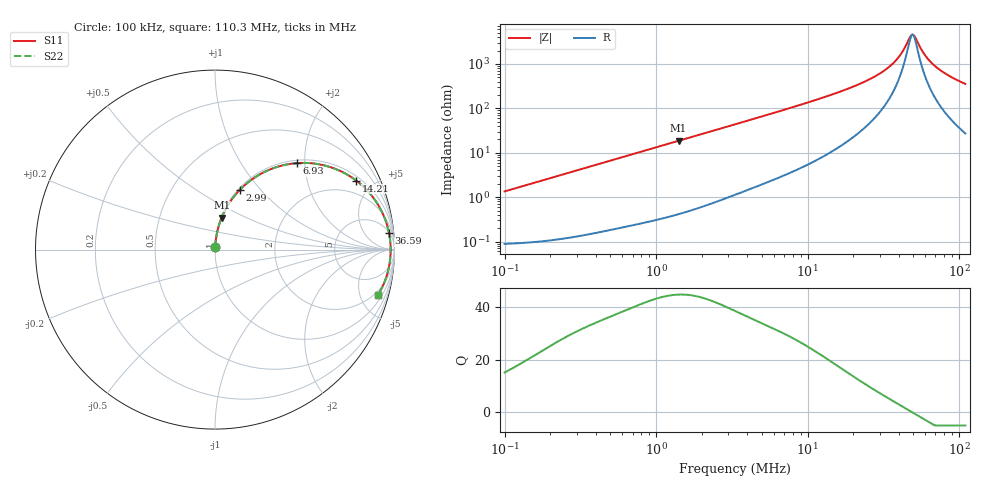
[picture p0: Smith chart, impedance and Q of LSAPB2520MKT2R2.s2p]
! LSAPB2520MKT2R2  S-PARAMETER MODEL  ( General Type )
! Model Generated by TAIYO YUDEN Corporation (http://www.ty-top.com)
! Version 2.0
! TAIYO YUDEN Control No. 20210629
! Copyright(c) 2015 TAIYO YUDEN CO.,LTD. All Rights Reserved.
! Product Description (link to TY-COMPAS)
! https://ds.yuden.co.jp/TYCOMPAS/or/detail?pn=LSAPB2520MKT2R2M&u=M
! Products Name : Inductors
! Characteristics :
!  Inductance : 2.2 uH , SRF(min) : -Hz , DC Resistance(max) : 0.09 Ohm
!  Rated Current : Saturation :2800 mA , Temp Rise : 2200 mA (40 degC)
!  Case Size : 2.5 x 2.0 / 0.098 x 0.079 [mm/inch] , Thickness : 1.2 / 0.047 [mm/inch]
!  (Conditions: Temperature = 25 degC , DC Bias Current/Voltage = 0A / 0V)
! External Node Assignments :
!  1  o---GGG---o  2
! GND o---------o GND
! Frequency Range : 0.1MHz  -  110.285862MHz  [ 402 STEP ]
# MHz S RI R 50
! Freq[MHz].  S11 Real  S11 Imag  S21 Real  S21 Imag  S12 Real  S12 Imag  S22 Real  S22 Imag
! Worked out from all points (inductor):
!   401 points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, 100 kHz to 110.3 MHz, reference 50 ohm
!   read as one part in series: L = 2.14 uH near 103.6 kHz
!   highest Q = 44.9 at 1.408 MHz (marker M1), where L = 2.1 uH
!   self-resonance near 49.28 MHz
!   S11 on the Smith chart (normalised r, x): 100 kHz: 1.00, +0.03; 2.99 MHz: 1.02, +0.79; 6.93 MHz: 1.06, +1.83; 14.21 MHz: 1.20, +3.98; 36.59 MHz: 6, +20; 110.3 MHz: 1.54, -7.08
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0.1  0.00107 0.0134  0.9989 -0.0134  0.9989 -0.0134  0.00107 0.0134
0.323312  0.00322 0.0431  0.9968 -0.0431  0.9968 -0.0431  0.00322 0.0431
1.045308  0.0217 0.1347  0.9783 -0.1347  0.9783 -0.1347  0.0217 0.1347
1.407833  0.037 0.178  0.963 -0.178  0.963 -0.178  0.037 0.178
2.989662  0.1397 0.3344  0.8603 -0.3344  0.8603 -0.3344  0.1397 0.3344
3.320932  0.1661 0.3594  0.8339 -0.3594  0.8339 -0.3594  0.1661 0.3594
4.71396  0.2827 0.4361  0.7173 -0.4361  0.7173 -0.4361  0.2827 0.4361
6.929861  0.4575 0.4819  0.5425 -0.4819  0.5425 -0.4819  0.4575 0.4819
10.73698  0.6722 0.449  0.3278 -0.449  0.3278 -0.449  0.6722 0.449
14.20963  0.7874 0.3843  0.2126 -0.3843  0.2126 -0.3843  0.7874 0.3843
24.031  0.9239 0.2228  0.0761 -0.2228  0.0761 -0.2228  0.9239 0.2228
29.65155  0.9525 0.1561  0.0475 -0.1561  0.0475 -0.1561  0.9525 0.1561
34.71395  0.9665 0.1071  0.0335 -0.1071  0.0335 -0.1071  0.9665 0.1071
36.58668  0.9699 0.0909  0.0301 -0.0909  0.0301 -0.0909  0.9699 0.0909
41.35872  0.9757 0.0536  0.0243 -0.0536  0.0243 -0.0536  0.9757 0.0536
47.57924  0.9786 0.0112  0.0214 -0.0112  0.0214 -0.0112  0.9786 0.0112
49.27539  0.9787 0.000661  0.0213 -0.000661  0.0213 -0.000661  0.9787 0.000661
51.03201  0.9787 -0.0099  0.0213 0.0099  0.0213 0.0099  0.9787 -0.0099
59.7447  0.9755 -0.0576  0.0245 0.0576  0.0245 0.0576  0.9755 -0.0576
68.73054  0.9685 -0.1005  0.0315 0.1005  0.0315 0.1005  0.9685 -0.1005
84.80576  0.9499 -0.1661  0.0501 0.1661  0.0501 0.1661  0.9499 -0.1661
110.2859  0.9101 -0.2504  0.0899 0.2504  0.0899 0.2504  0.9101 -0.2504
